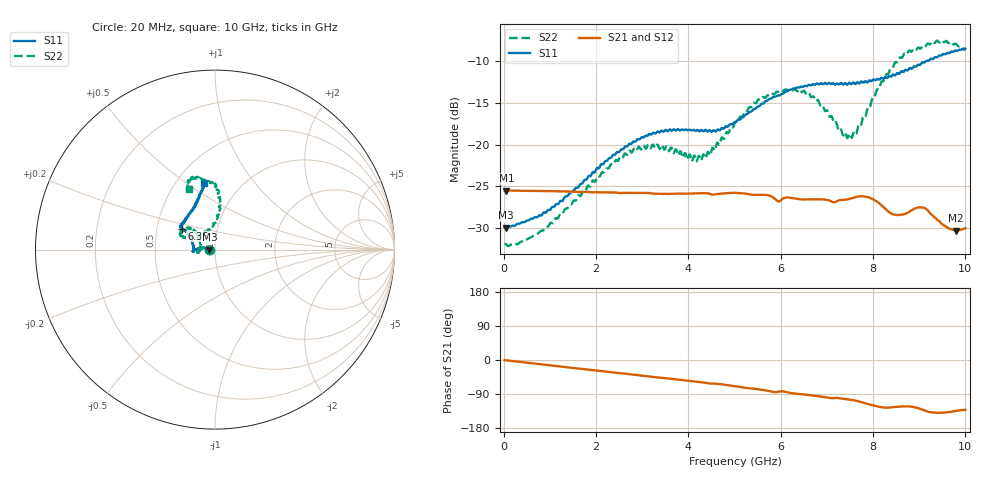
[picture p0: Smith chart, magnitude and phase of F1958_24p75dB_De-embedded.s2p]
! Integrated Device Technology
! Corporate Headquarters
! 6024 Silver Creek Valley Road
! San Jose, CA 95138  USA
! Phone:  1-408-284-8200
! Toll Free:  1-800-223-1366
! Webpage:  http://www.idt.com/
! Timing and RF Division
! 515 Groton Road, Suite 102
! Westford, MA 01886-6024
! Device:  F1958
! Description: 7-bit 0.25 dB Digital Step Attenuator
! Frequency:  0.001 -  6.000 GHz
! Package:  4x4 mm Thin QFN Plastic Package: 24 pin
! Ports:  2 RF, 12 DC
!  Pin  1  = D0
!  Pin  2  = VDD
!  Pin  3  = VMODE
!  Pin  4  = GND
!  Pin  5  = RF1  =  Port 1
!  Pin  6  = GND
!  Pin  7  = GND
!  Pin  8  = GND
!  Pin  9  = GND
!  Pin 10  = GND
!  Pin 11  = GND
!  Pin 12  = GND
!  Pin 13  = GND
!  Pin 14  = RF2  =  Port 2
!  Pin 15  = GND
!  Pin 16  = LE
!  Pin 17  = CLK
!  Pin 18  = DATA
!  Pin 19  = D6
!  Pin 20  = D5
!  Pin 21  = D4
!  Pin 22  = D3
!  Pin 23  = D2
!  Pin 24  = D1
! State:  99
! Atten State:  24.75 dB
! Voltage:  +3.30 Volts
! Current:  0.258 mA
! Data:  The device was measured on a F1958 evaluation board which has
!  individual transmission lines to the RF pins.  Data was collected
!  using a calibrated network analyzer.  The evaluation board was
!  de-embedded using Automatic Fixture Removal (AFR).
!  The reference plane is the edge of the package pin.
! Misc:
!  Action Tracker AT0419
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# GHz S dB R 50
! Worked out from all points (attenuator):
!   500 points, 20 MHz to 10 GHz, reference 50 ohm
!   highest |S21| = -25.54 dB at 60 MHz (marker M1); lowest = -30.4 dB at 9.8 GHz (marker M2)
!   lowest |S11| = -30.0 dB at 40 MHz (marker M3), VSWR 1.07, Z = 46.9 - j0.0427 ohm
!   |S11| at or under -10 dB: start of sweep to 9.14 GHz
!   |S22| runs from -32.2 to -7.5 dB; largest |S21 - S12| = 0.00024
!   S11 on the Smith chart (normalised r, x): 20 MHz: 0.94, -0.00; 6.38 GHz: 0.67, +0.17; 10 GHz: 0.68, +0.59
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0.02  -29.98 -178.9  -25.55 -0.3  -25.54 -0.3  -32.01 -178.9
0.04  -30.00 -179.2  -25.54 -0.6  -25.54 -0.5  -31.98 -178.3
0.06  -29.99 179.9  -25.54 -0.9  -25.54 -0.8  -32.05 -178.3
0.84  -28.39 171.3  -25.61 -11.8  -25.59 -11.7  -30.38 172.9
1.7  -24.72 171.2  -25.72 -23.5  -25.72 -23.4  -25.76 171.9
2.62  -20.30 177.1  -25.83 -36.0  -25.81 -36.0  -21.09 -179.3
3.36  -18.53 -175.8  -25.93 -46.3  -25.92 -46.4  -20.35 -169.6
4.24  -18.42 -179.3  -25.87 -58.0  -25.88 -58.1  -21.41 168.7
4.5  -18.48 174.8  -26.02 -62.3  -26.03 -62.2  -20.77 151.5
5.02  -17.34 160.5  -25.81 -69.3  -25.83 -69.3  -17.26 138.3
5.58  -15.11 150.3  -26.07 -78.3  -26.08 -78.3  -14.56 139.8
6.38  -13.14 147.8  -26.57 -89.6  -26.59 -89.5  -13.49 154.6
6.68  -12.78 146.3  -26.59 -93.3  -26.61 -93.2  -14.26 157.2
7.32  -12.61 141.0  -26.68 -102.0  -26.68 -101.8  -18.39 138.7
7.5  -12.61 137.9  -26.55 -104.6  -26.55 -104.5  -18.71 119.2
7.68  -12.57 134.9  -26.26 -109.0  -26.25 -108.9  -17.77 99.6
7.9  -12.38 128.5  -26.35 -116.5  -26.36 -116.6  -15.52 89.4
8.34  -11.78 118.6  -28.10 -125.6  -28.10 -125.7  -11.39 83.9
8.66  -11.28 112.9  -28.42 -122.4  -28.40 -122.3  -9.21 87.5
9.1  -10.12 106.7  -27.62 -132.3  -27.62 -132.4  -8.10 100.0
9.8  -8.68 100.3  -30.36 -134.2  -30.37 -134.3  -7.88 112.3
10  -8.48 99.5  -30.06 -131.4  -30.12 -131.3  -8.64 113.3
